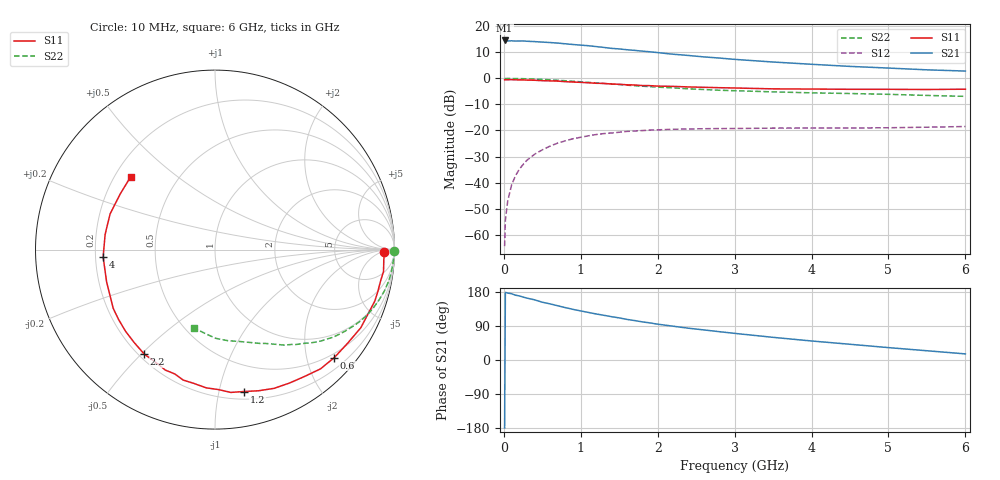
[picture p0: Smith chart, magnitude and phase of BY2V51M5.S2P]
! SIEMENS Small Signal Semiconductors
! BFY420
! Si NPN RF SIEGET Grounded Emitter Transistor in MICRO-X
! VCE = 2.5 V  IC = 1.5 mA
! Common Emitter S-Parameters:  October  1996
# GHz  S  MA  R  50
!  f  S11  S21  S12  S22
! GHz  MAG  ANG  MAG  ANG  MAG  ANG  MAG  ANG
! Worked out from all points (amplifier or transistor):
!   36 points, 10 MHz to 6 GHz, reference 50 ohm
!   highest |S21| = 14.6 dB at 10 MHz (marker M1)
!   |S21| within 3 dB of that: start of sweep to 1.389 GHz
!   unconditionally stable (mu >= 1): 4.274 GHz to end of sweep
!   at 250 MHz: K = 0.05, MSG = 23.7 dB, |S12| = -33.1 dB
!   at 1.4 GHz: K = 0.25, MSG = 16.3 dB, |S12| = -21.0 dB
!   at 6 GHz: K = 1.29, MAG = 7.4 dB, |S12| = -18.5 dB
!   S11 on the Smith chart (normalised r, x): 10 MHz: 31, -8; 600 MHz: 0.41, -2.53; 1.2 GHz: 0.26, -1.19; 2.2 GHz: 0.22, -0.51; 4 GHz: 0.23, -0.03; 6 GHz: 0.26, +0.35
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0.01  0.9419 -0.9  5.357 -179.4  0.0006 97.2  0.9983 -0.4
0.02  0.9432 -1.7  5.344 178.5  0.0019 92.2  0.993 -0.7
0.05  0.9422 -3.4  5.239 176.7  0.0044 87.6  0.9972 -1.8
0.1  0.9469 -7.4  5.276 174.9  0.0089 84.2  0.9957 -3.5
0.15  0.9389 -10.7  5.217 171.1  0.0134 83.8  0.993 -5.2
0.25  0.9355 -17.8  5.238 166.1  0.0222 78.7  0.9871 -8.7
0.4  0.9216 -28.2  5.094 158.7  0.035 73.0  0.9712 -13.8
0.5  0.9044 -35.3  4.98 152.5  0.0425 69.6  0.956 -17.1
0.6  0.8965 -42.2  4.891 148.1  0.0501 65.6  0.9397 -20.3
0.8  0.8657 -54.6  4.619 138.2  0.0633 58.0  0.9016 -26.3
1.1  0.823 -72.9  4.245 125.5  0.079 48.5  0.8392 -34.1
1.2  0.8071 -78.4  4.086 121.5  0.0836 45.4  0.8199 -36.5
1.6  0.7545 -99.1  3.552 107.1  0.096 35.9  0.7421 -44.5
2  0.7115 -116.8  3.131 94.5  0.103 28.1  0.6798 -51.0
2.2  0.7029 -124.2  2.916 89.2  0.1054 24.9  0.6577 -54.0
2.4  0.6858 -131.2  2.758 83.9  0.1068 22.4  0.6305 -56.9
2.8  0.6634 -144.1  2.462 74.7  0.1088 17.9  0.5925 -61.9
3.5  0.63 -163.5  2.064 59.8  0.1109 12.6  0.5512 -69.7
4  0.6245 -176.2  1.868 50.2  0.1113 10.4  0.5281 -75.6
4.5  0.618 172.2  1.701 41.5  0.1116 8.6  0.5127 -81.9
5.5  0.6123 149.6  1.461 24.4  0.1157 7.6  0.471 -96.6
6  0.6207 139.3  1.384 16.1  0.1192 7.7  0.4521 -104.9
